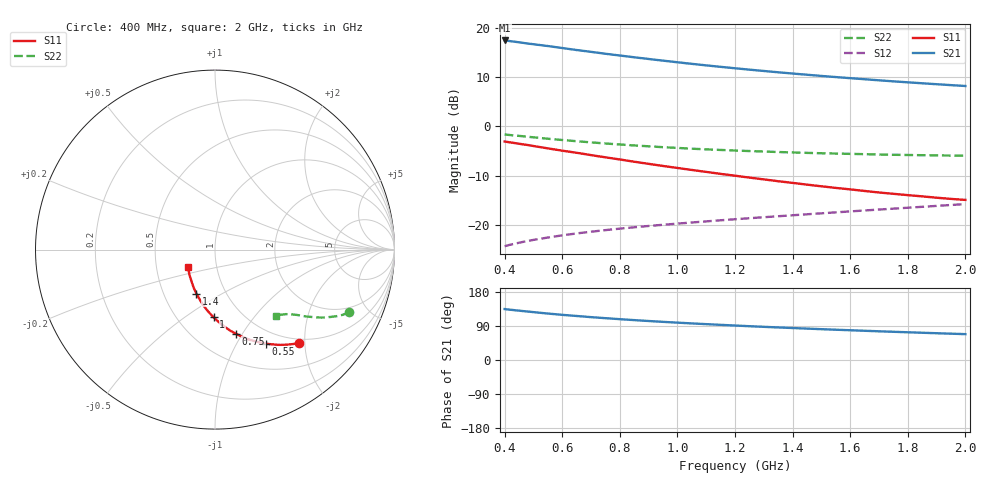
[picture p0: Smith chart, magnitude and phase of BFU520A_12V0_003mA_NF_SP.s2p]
! Filename:  P:\Prog\Test\Noise\ATS_data\Testdata_Net\06 Compressed Noise after Statistics\BFU520A_APG2013_30_A05_12p0V_003mA_NF_CM01_D.sf
! Date/Time: Wed 24/Apr/2013 20:06:21
! BFU520A_APG2013_30_A05_12p0V_1to20mA_NF_CM01_Bias3_R.sf
! Noise Parameter Data File
! BFU520A_APG2013_30_A05_12p0V_1to20mA_NF_CM01
! Date/time: Thu Apr 11 10:46:45 2013
! VAR V_out= 12.001000
! VAR I_out= 3.000000
! VAR V_in= 0.809700
! VAR I_in= 0.028605
! Device data file deembeded for feedlines and parallel
! Original file: \06 Compressed Noise after Statistics\BFU520A_APG2013_30_A05_12p0V_003mA_NF_CM01_R.sf
! Feed-files: PR017V01_150413_Feed1.s2p, PR017V01_150413_Feed2.s2p
! Parallel-file: PR017V01_150413_Par.s2p
# MHz S MA R 50
!  Freq-MHz  S11-mag  S11-arg  S21-mag  S21-arg  S12-mag  S12-arg  S22-mag  S22-arg
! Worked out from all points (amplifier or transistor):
!   37 points, 400 MHz to 2 GHz, reference 50 ohm
!   highest |S21| = 17.5 dB at 400 MHz (marker M1)
!   |S21| within 3 dB of that: start of sweep to 791.3 MHz
!   unconditionally stable (mu >= 1): 1.926 GHz to end of sweep
!   at 500 MHz: K = 0.46, MSG = 19.9 dB, |S12| = -23.1 dB
!   at 1.1 GHz: K = 0.81, MSG = 15.9 dB, |S12| = -19.3 dB
!   at 2 GHz: K = 1.01, MAG = 11.6 dB, |S12| = -15.8 dB
!   lowest NFmin = 0.56 dB at 420 MHz
!   S11 on the Smith chart (normalised r, x): 400 MHz: 0.92, -1.89; 550 MHz: 0.82, -1.34; 750 MHz: 0.77, -0.94; 1 GHz: 0.74, -0.65; 1.4 GHz: 0.73, -0.38; 2 GHz: 0.73, -0.15
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400  0.7008 -47.9  7.468 134.4  0.06047 65.2  0.8258 -25.1
420  0.6864 -49.9  7.346 132.7  0.06261 64.5  0.8151 -25.9
460  0.6585 -53.6  7.087 129.4  0.06646 63.2  0.7945 -27.3
500  0.6309 -57.1  6.837 126.3  0.07005 62.1  0.7735 -28.6
550  0.5971 -61.5  6.554 122.6  0.07404 60.9  0.748 -30.1
600  0.5656 -65.4  6.256 119.2  0.0779 60.0  0.7262 -31.3
650  0.5385 -68.9  5.97 116.2  0.08149 59.2  0.706 -32.4
700  0.5099 -72.6  5.722 113.1  0.08483 58.6  0.6869 -33.4
750  0.4841 -75.8  5.47 110.4  0.08805 58.2  0.6696 -34.2
800  0.4605 -79.2  5.249 107.8  0.09114 57.9  0.6537 -35.0
850  0.4367 -82.4  5.037 105.2  0.09412 57.6  0.6393 -35.8
900  0.4157 -85.4  4.84 102.9  0.09704 57.4  0.6265 -36.4
950  0.3953 -88.3  4.655 100.7  0.09976 57.4  0.6137 -37.0
1000  0.3775 -91.1  4.481 98.6  0.1025 57.3  0.6032 -37.6
1100  0.3442 -96.8  4.167 94.6  0.108 57.5  0.5835 -38.6
1200  0.3149 -102.3  3.895 91.0  0.1136 57.7  0.5674 -39.6
1300  0.2888 -107.5  3.656 87.5  0.1191 58.0  0.5544 -40.6
1400  0.2661 -112.9  3.442 84.4  0.1247 58.5  0.5428 -41.5
1500  0.2457 -118.4  3.254 81.3  0.1305 58.9  0.5326 -42.5
1650  0.2203 -126.5  3.012 77.1  0.1395 59.5  0.5212 -44.0
1750  0.206 -132.4  2.867 74.4  0.1456 59.9  0.5138 -45.0
2000  0.1786 -146.9  2.571 68.2  0.162 60.8  0.5021 -47.8
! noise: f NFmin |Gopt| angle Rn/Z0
400  0.6221  0.3801  13.95  0.1771
460  0.6267  0.3588  17.35  0.1641
600  0.6652  0.3686  20.24  0.1965
800  0.6783  0.3416  36.11  0.1488
1000  0.7304  0.3225  47  0.1358
1200  0.7448  0.3034  56.71  0.1383
1400  0.7671  0.2947  72.42  0.1234
1600  0.806  0.2544  80.22  0.1124
1800  0.7495  0.2294  102.8  0.0936
2000  0.7697  0.2093  110.7  0.0965
